FUNCTION "C TAVOLA" : VOID
TITLE =CICLO TAVOLA
VERSION : 0.1

BEGIN
NETWORK
TITLE =ATTESA START
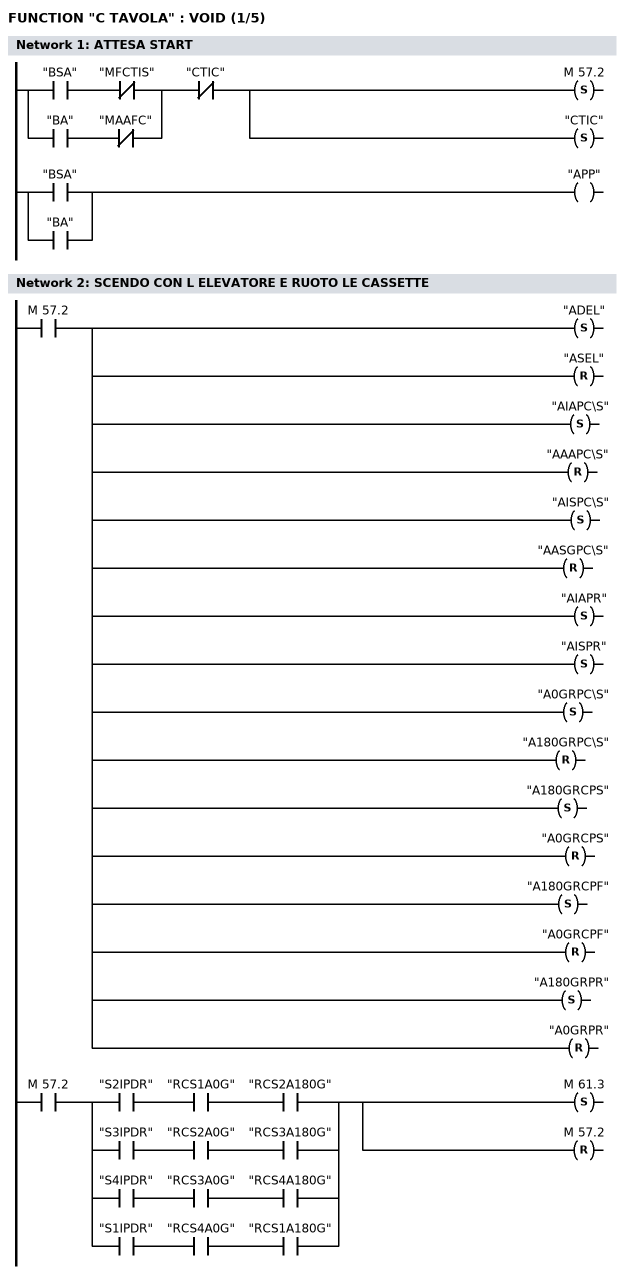
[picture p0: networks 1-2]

      U(    ;
      U     "BSA";
      UN    "MFCTIS";
      O     ;
      U     "BA";
      UN    "MAAFC";
      )     ;
      UN    "CTIC";
      S     M     57.2;
      S     "CTIC";

      U(    ;
      U     "BSA";
      O     "BA";
      )     ;
      =     "APP";
NETWORK
TITLE =SCENDO CON L ELEVATORE E RUOTO LE CASSETTE

      U     M     57.2;
      S     "ADEL";
      R     "ASEL";
      S     "AIAPC\S";
      R     "AAAPC\S";
      S     "AISPC\S";
      R     "AASGPC\S";
      S     "AIAPR";
      S     "AISPR";
      S     "A0GRPC\S";
      R     "A180GRPC\S";
      S     "A180GRCPS";
      R     "A0GRCPS";
      S     "A180GRCPF";
      R     "A0GRCPF";
      S     "A180GRPR";
      R     "A0GRPR";

      U     M     57.2;
      U(    ;
      U     "S2IPDR";
      U     "RCS1A0G";
      U     "RCS2A180G";
      O     ;
      U     "S3IPDR";
      U     "RCS2A0G";
      U     "RCS3A180G";
      O     ;
      U     "S4IPDR";
      U     "RCS3A0G";
      U     "RCS4A180G";
      O     ;
      U     "S1IPDR";
      U     "RCS4A0G";
      U     "RCS1A180G";
      )     ;
      S     M     61.3;
      R     M     57.2;
NETWORK
TITLE =VERIFICO ELEVATORE LIBERO
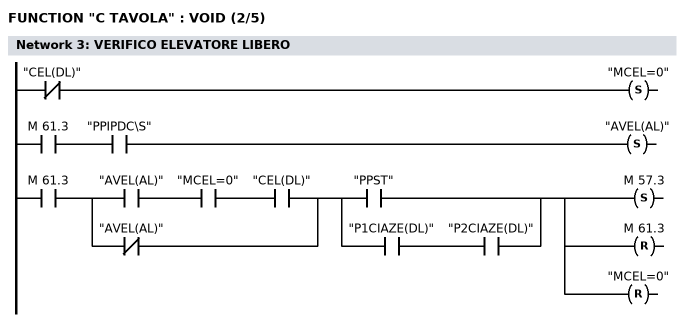
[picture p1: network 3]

      UN    "CEL(DL)";
      S     "MCEL=0";

      U     M     61.3;
      U     "PPIPDC\S";
      S     "AVEL(AL)";

      U     M     61.3;
      U(    ;
      U     "AVEL(AL)";
      U     "MCEL=0";
      U     "CEL(DL)";
      O     ;
      UN    "AVEL(AL)";
      )     ;
      U(    ;
      U     "PPST";
      O     ;
      U     "P1CIAZE(DL)";
      U     "P2CIAZE(DL)";
      )     ;
      S     M     57.3;
      R     M     61.3;
      R     "MCEL=0";
NETWORK
TITLE =START CICLI
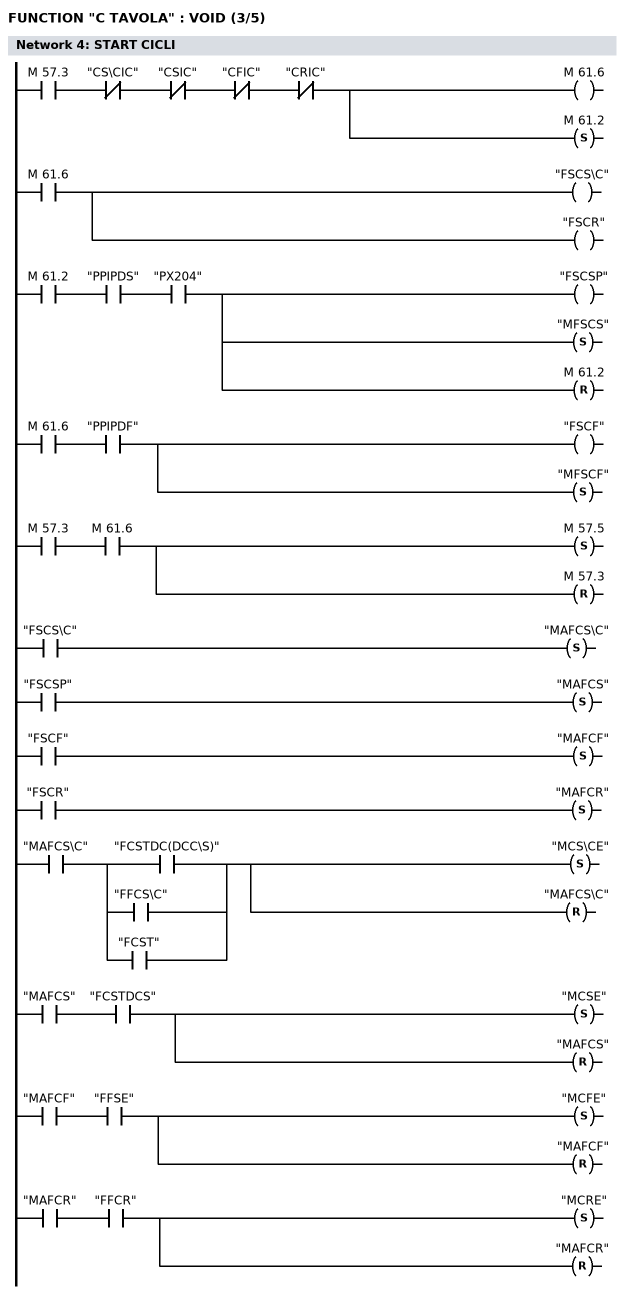
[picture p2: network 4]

      U     M     57.3;
      UN    "CS\CIC";
      UN    "CSIC";
      UN    "CFIC";
      UN    "CRIC";
      =     M     61.6;
      S     M     61.2;
      U     M     61.6;
      =     "FSCS\C";
      =     "FSCR";
      U     M     61.2;
      U     "PPIPDS";
      U     "PX204";
      =     "FSCSP";
      S     "MFSCS";
      R     M     61.2;
      U     M     61.6;
      U     "PPIPDF";
      =     "FSCF";
      S     "MFSCF";

      U     M     57.3;
      U     M     61.6;
      S     M     57.5;
      R     M     57.3;

      U     "FSCS\C";
      S     "MAFCS\C";

      U     "FSCSP";
      S     "MAFCS";

      U     "FSCF";
      S     "MAFCF";

      U     "FSCR";
      S     "MAFCR";

      U     "MAFCS\C";
      U(    ;
      U     "FCSTDC(DCC\S)";
      O     "FFCS\C";
      O     "FCST";
      )     ;
      S     "MCS\CE";
      R     "MAFCS\C";

      U     "MAFCS";
      U     "FCSTDCS";
      S     "MCSE";
      R     "MAFCS";

      U     "MAFCF";
      U     "FFSE";
      S     "MCFE";
      R     "MAFCF";

      U     "MAFCR";
      U     "FFCR";
      S     "MCRE";
      R     "MAFCR";
NETWORK
TITLE =ATTESA TEMPO COLATA
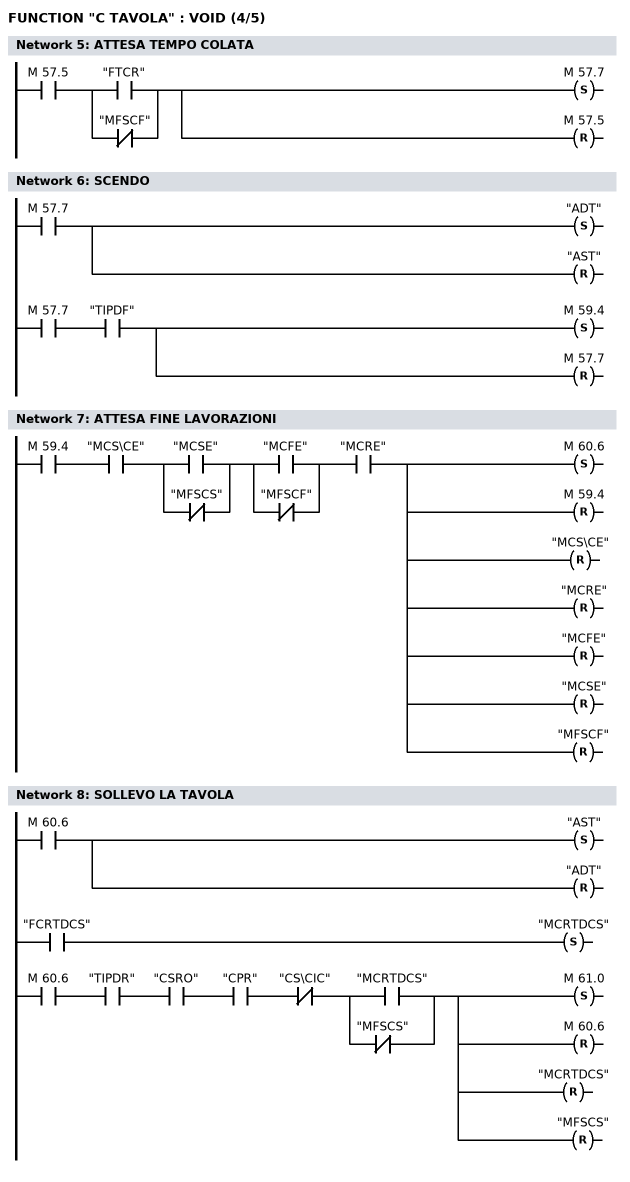
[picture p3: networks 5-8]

      U     M     57.5;
      U(    ;
      O     "FTCR";
      ON    "MFSCF";
      )     ;
      S     M     57.7;
      R     M     57.5;
NETWORK
TITLE =SCENDO

      U     M     57.7;
      S     "ADT";
      R     "AST";

      U     M     57.7;
      U     "TIPDF";
      S     M     59.4;
      R     M     57.7;
NETWORK
TITLE =ATTESA FINE LAVORAZIONI

      U     M     59.4;
      U     "MCS\CE";
      U(    ;
      O     "MCSE";
      ON    "MFSCS";
      )     ;
      U(    ;
      O     "MCFE";
      ON    "MFSCF";
      )     ;
      U     "MCRE";
      S     M     60.6;
      R     M     59.4;
      R     "MCS\CE";
      R     "MCRE";
      R     "MCFE";
      R     "MCSE";
      R     "MFSCF";
NETWORK
TITLE =SOLLEVO LA TAVOLA

      U     M     60.6;
      S     "AST";
      R     "ADT";

      U     "FCRTDCS";
      S     "MCRTDCS";

      U     M     60.6;
      U     "TIPDR";
      U     "CSRO";
      U     "CPR";
      UN    "CS\CIC";
      U(    ;
      U     "MCRTDCS";
      ON    "MFSCS";
      )     ;
      S     M     61.0;
      R     M     60.6;
      R     "MCRTDCS";
      R     "MFSCS";
NETWORK
TITLE =RUOTO LA TAVOLA
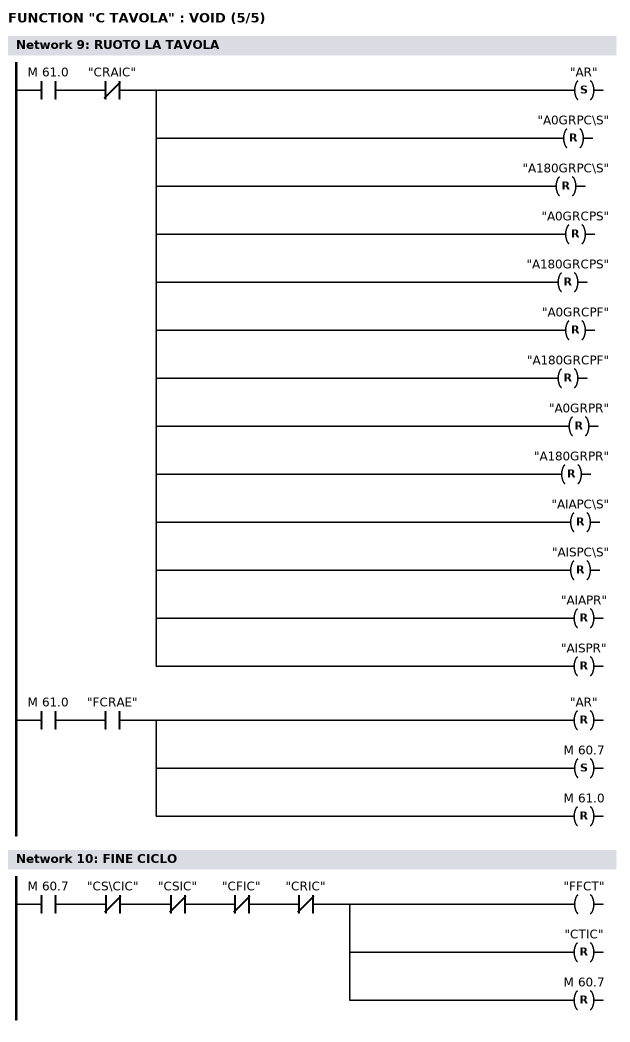
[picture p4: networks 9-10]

      U     M     61.0;
      UN    "CRAIC";
      S     "AR";
      R     "A0GRPC\S";
      R     "A180GRPC\S";
      R     "A0GRCPS";
      R     "A180GRCPS";
      R     "A0GRCPF";
      R     "A180GRCPF";
      R     "A0GRPR";
      R     "A180GRPR";
      R     "AIAPC\S";
      R     "AISPC\S";
      R     "AIAPR";
      R     "AISPR";

      U     M     61.0;
      U     "FCRAE";
      R     "AR";
      S     M     60.7;
      R     M     61.0;
NETWORK
TITLE =FINE CICLO

      U     M     60.7;
      UN    "CS\CIC";
      UN    "CSIC";
      UN    "CFIC";
      UN    "CRIC";
      =     "FFCT";
      R     "CTIC";
      R     M     60.7;
NETWORK
TITLE =RESET CICLO

      U     "BRA";
      SPBN  RES;
      L     0;
      T     MB    57;
      T     MB    59;
      T     MB    60;
      T     MB    61;
      SET   ;
      R     "A0GRPC\S";
      R     "A180GRPC\S";
      R     "A180GRCPS";
      R     "A0GRCPS";
      R     "A180GRCPF";
      R     "A0GRCPF";
      R     "A0GRPR";
      R     "A180GRPR";
      R     "AST";
      R     "ADT";
      R     "AR";
      R     "AVEL(AL)";
RES:  NOP   0;
END_FUNCTION

